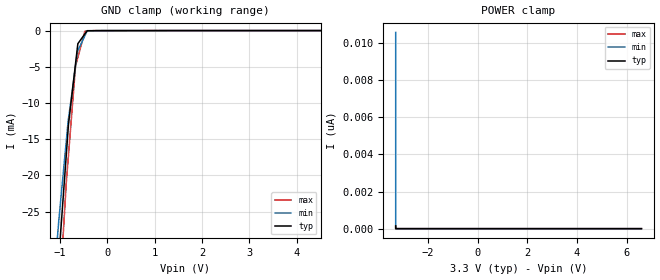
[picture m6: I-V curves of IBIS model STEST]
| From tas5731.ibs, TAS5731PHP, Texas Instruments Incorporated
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[Model]   STEST
Model_type   Input
Vinl = .8
Vinh = 2
|   typ   min   max
C_comp   0.7443p   0.7440p   0.7473p
[Voltage Range]   3.3   3   3.6
[Temperature Range]   27   125   0
[Power Clamp Reference]   3.3   3   3.6
[GND Clamp Reference]   -0   -0   -0
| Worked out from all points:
|   GND clamp passes 1 mA (typ) near -0.53 V on its own axis
[GND Clamp]
|   Voltage   I(typ)   I(min)   I(max)
-3.3V     -1.546A    -1.399A    -1.589A
-1.063V   -36.08mA   -29.7mA    -43.4mA
-1.022V   -31.68mA   -26.36mA   -38.78mA
-1.014V   -30.86mA   -25.82mA   -37.92mA
-865.4mV  -17.41mA   -15.44mA   -21.23mA
-816.4mV  -12.99mA   -12.19mA   -17.19mA
-667.4mV  -4.573mA   -4.904mA   -4.892mA
-618.4mV  -1.807mA   -2.778mA   -3.705mA
-469.4mV  -459.7uA   -687.7uA   -90.19uA
-428.1mV  -86.38uA   -108.7uA   -71.41uA
-230.1mV  -15.53uA   -915.6nA   -82.61nA
6.6V      0A         0A         0A
[POWER Clamp]
|   Voltage   I(typ)   I(min)   I(max)
-3.3V     150.4pA    10.58nA    123.2pA
-3.3V     0A         0A         0A
-3.3V     0A         0A         0A
6.6V      0A         0A         0A
